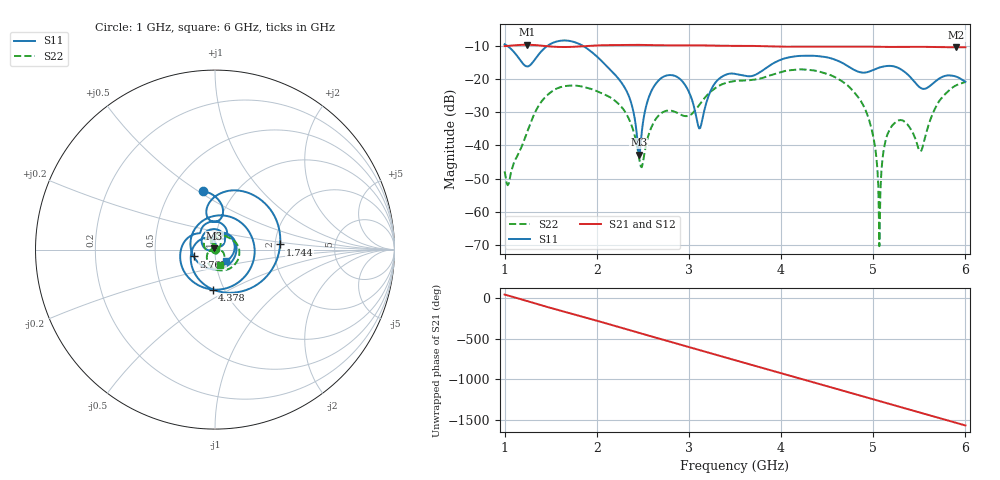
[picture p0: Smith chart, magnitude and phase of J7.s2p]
!Agilent Technologies,E8364B,MY43040528,A.07.50.67
!Agilent E8364B: A.07.50.67
!Date: Sunday, March 01, 2026 18:28:34
!Correction: S11(Full 2 Port(1,2))
!S21(Full 2 Port(1,2))
!S12(Full 2 Port(1,2))
!S22(Full 2 Port(1,2))
!S2P File: Measurements: S11, S21, S12, S22:
# Hz S  dB  R 50
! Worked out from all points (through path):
!   451 points, 1 GHz to 6 GHz, reference 50 ohm
!   highest |S21| = -9.67 dB at 1.244 GHz (marker M1); lowest = -10.4 dB at 5.9 GHz (marker M2)
!   group delay of S21, straight-line fit = 896 ps
!   lowest |S11| = -42.8 dB at 2.456 GHz (marker M3), VSWR 1.01, Z = 49.7 + j0.646 ohm
!   |S11| at or under -10 dB: 1.028 GHz to 1.466 GHz (437.6 MHz wide, 35.1 % of centre); 1.849 GHz to end of sweep
!   |S22| runs from -70.4 to -17.1 dB; largest |S21 - S12| = 0.0013
!   S11 on the Smith chart (normalised r, x): 1 GHz: 0.71, +0.52; 1.744 GHz: 2.13, +0.14; 3.767 GHz: 0.78, -0.06; 4.378 GHz: 0.88, -0.41; 6 GHz: 1.12, -0.15
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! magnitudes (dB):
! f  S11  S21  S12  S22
! 1 GHz  -9.5  -10.1  -10.1  -47.8
! 1.244 GHz  -16.2  -9.7  -9.7  -36.0
! 1.744 GHz  -8.8  -10.3  -10.3  -22.0
! 1.844 GHz  -9.9  -10.1  -10.2  -22.3
! 2.311 GHz  -23.0  -9.7  -9.8  -30.1
! 2.456 GHz  -42.8  -9.7  -9.7  -43.1
! 2.667 GHz  -20.6  -9.8  -9.8  -31.1
! 2.922 GHz  -20.5  -9.9  -9.9  -30.9
! 3.111 GHz  -34.9  -9.9  -9.9  -27.8
! 3.278 GHz  -21.4  -9.9  -10.0  -22.9
! 3.5 GHz  -18.4  -10.0  -10.0  -20.6
! 3.767 GHz  -18.0  -10.1  -10.1  -19.9
! 4.344 GHz  -13.0  -10.2  -10.3  -17.4
! 4.378 GHz  -13.0  -10.2  -10.3  -17.5
! 4.889 GHz  -18.1  -10.2  -10.2  -27.8
! 5 GHz  -17.3  -10.3  -10.3  -37.3
! 5.067 GHz  -16.5  -10.3  -10.3  -70.4
! 5.167 GHz  -16.0  -10.3  -10.4  -35.9
! 5.322 GHz  -17.5  -10.3  -10.4  -32.5
! 5.511 GHz  -22.6  -10.3  -10.3  -41.8
! 5.9 GHz  -19.3  -10.4  -10.5  -21.9
! 6 GHz  -20.8  -10.4  -10.4  -20.9
